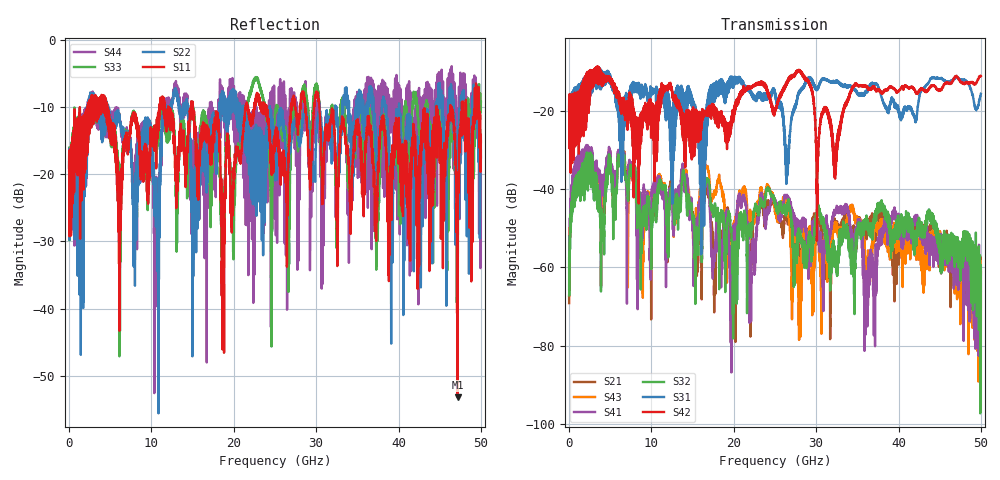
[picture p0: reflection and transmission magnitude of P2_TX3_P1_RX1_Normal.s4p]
!Keysight Technologies,N5225B,MY57041031,A.13.20.10
!Date: Friday, May 31, 2019 11:14:42
!Correction: S11(Full 4 Port(1,2,3,4))
!S12(Full 4 Port(1,2,3,4))
!S13(Full 4 Port(1,2,3,4))
!S14(Full 4 Port(1,2,3,4))
!S21(Full 4 Port(1,2,3,4))
!S22(Full 4 Port(1,2,3,4))
!S23(Full 4 Port(1,2,3,4))
!S24(Full 4 Port(1,2,3,4))
!S31(Full 4 Port(1,2,3,4))
!S32(Full 4 Port(1,2,3,4))
!S33(Full 4 Port(1,2,3,4))
!S34(Full 4 Port(1,2,3,4))
!S41(Full 4 Port(1,2,3,4))
!S42(Full 4 Port(1,2,3,4))
!S43(Full 4 Port(1,2,3,4))
!S44(Full 4 Port(1,2,3,4))
!S4P File: Measurements: <S11,S12,S13,S14>,
!<S21,S22,S23,S24>,
!<S31,S32,S33,S34>,
!<S41,S42,S43,S44>:
# Hz S  dB  R 50.0
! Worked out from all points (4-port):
!   5000 points, 10 MHz to 50 GHz, reference 50 ohm
!   strongest paths, dB at 10 MHz, 12.51 GHz, 25.01 GHz, 37.51 GHz, 50 GHz:
!     S42: -19.5, -14.7, -19.8, -14.6, -11.1
!     S31: -19.6, -43.0, -16.0, -13.6, -15.6
!     S32: -57.8, -38.8, -44.1, -45.5, -61.3
!     S41: -65.6, -42.4, -43.0, -53.3, -65.7
!     S43: -67.2, -41.6, -45.5, -49.1, -60.6
!     S21: -69.2, -37.1, -44.8, -47.6, -66.4
!   lowest |S11| = -53.1 dB at 47.18 GHz (marker M1), VSWR 1.00, Z = 49.8 - j0.0965 ohm
!   |S11| at or under -10 dB: 4.63 GHz to 10.95 GHz (6.318 GHz wide, 81.1 % of centre); 15.04 GHz to 21.46 GHz (6.426 GHz wide, 35.2 % of centre); 30.38 GHz to 44.61 GHz (14.23 GHz wide, 37.9 % of centre)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
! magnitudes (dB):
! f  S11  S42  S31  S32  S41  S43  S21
! 10 MHz  -19.5  -19.5  -19.6  -57.8  -65.6  -67.2  -69.2
! 6.45 GHz  -18.4  -19.6  -25.9  -30.5  -29.8  -30.1  -29.6
! 21.93 GHz  -11.4  -13.7  -14.9  -49.9  -57.6  -45.9  -67.5
! 24.68 GHz  -17.5  -18.6  -14.5  -41.7  -41.9  -41.1  -43.4
! 28 GHz  -11.2  -9.6  -14.8  -52.6  -49.0  -67.6  -58.1
! 47.18 GHz  -53.1  -11.4  -11.4  -52.3  -61.1  -59.0  -56.6
! 50 GHz  -15.3  -11.1  -15.6  -61.3  -65.7  -60.6  -66.4
